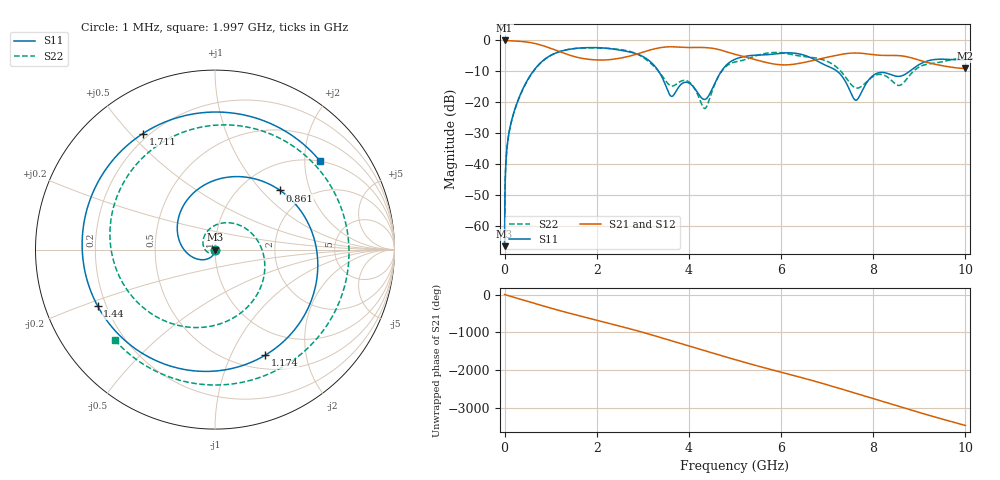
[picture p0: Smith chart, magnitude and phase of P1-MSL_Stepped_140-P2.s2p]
!Created with skrf (http://scikit-rf.org).
# GHz S RI R 50.0
!freq ReS11 ImS11 ReS21 ImS21 ReS12 ImS12 ReS22 ImS22
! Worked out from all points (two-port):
!   10000 points, 1 MHz to 10 GHz, reference 50 ohm
!   highest |S21| = 0.00 dB at 1 MHz (marker M1); lowest = -9.1 dB at 10 GHz (marker M2)
!   |S21| within 3 dB of the highest: start of sweep to 1.081 GHz; 3.176 GHz to 4.663 GHz (1.486 GHz wide, 37.9 % of centre)
!   lowest |S11| = -66.5 dB at 1 MHz (marker M3), VSWR 1.00, Z = 50 - j0.0474 ohm
!   |S11| at or under -10 dB: start of sweep to 619 MHz; 3.345 GHz to 4.703 GHz (1.357 GHz wide, 33.7 % of centre); 7.221 GHz to 8.786 GHz (1.566 GHz wide, 19.6 % of centre)
!   |S22| runs from -66.5 to -2.4 dB; largest |S21 - S12| = 7e-16
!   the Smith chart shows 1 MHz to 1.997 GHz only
!   S11 on the Smith chart (normalised r, x): 1 MHz: 1.00, -0.00; 861 MHz: 1.48, +1.28; 1.174 GHz: 0.67, -1.36; 1.44 GHz: 0.17, -0.22; 1.711 GHz: 0.18, +0.54; 1.997 GHz: 0.99, +2.36
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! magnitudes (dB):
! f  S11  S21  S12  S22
! 1 MHz  -66.5  0.0  0.0  -66.5
! 63 MHz  -33.3  -0.1  -0.1  -33.4
! 170 MHz  -24.9  -0.1  -0.1  -25.0
! 473 MHz  -13.4  -0.5  -0.5  -13.6
! 861 MHz  -6.2  -1.8  -1.8  -6.3
! 1.174 GHz  -3.7  -3.5  -3.5  -3.7
! 1.44 GHz  -2.8  -4.9  -4.9  -2.8
! 1.668 GHz  -2.4  -5.7  -5.7  -2.5
! 1.711 GHz  -2.4  -5.9  -5.9  -2.5
! 1.997 GHz  -2.3  -6.3  -6.3  -2.5
! 3.334 GHz  -9.7  -2.5  -2.5  -9.8
! 3.61 GHz  -18.0  -2.0  -2.0  -14.7
! 3.994 GHz  -13.7  -2.3  -2.3  -13.3
! 4.346 GHz  -19.0  -2.3  -2.3  -22.0
! 4.689 GHz  -10.3  -3.1  -3.1  -10.4
! 5.001 GHz  -6.1  -4.5  -4.5  -7.0
! 6.667 GHz  -5.7  -6.6  -6.6  -5.5
! 7.252 GHz  -10.4  -4.7  -4.7  -9.3
! 7.617 GHz  -19.3  -4.1  -4.1  -15.3
! 7.994 GHz  -11.4  -4.6  -4.6  -11.7
! 8.334 GHz  -10.8  -4.8  -4.8  -12.1
! 10 GHz  -6.2  -9.1  -9.1  -5.8
